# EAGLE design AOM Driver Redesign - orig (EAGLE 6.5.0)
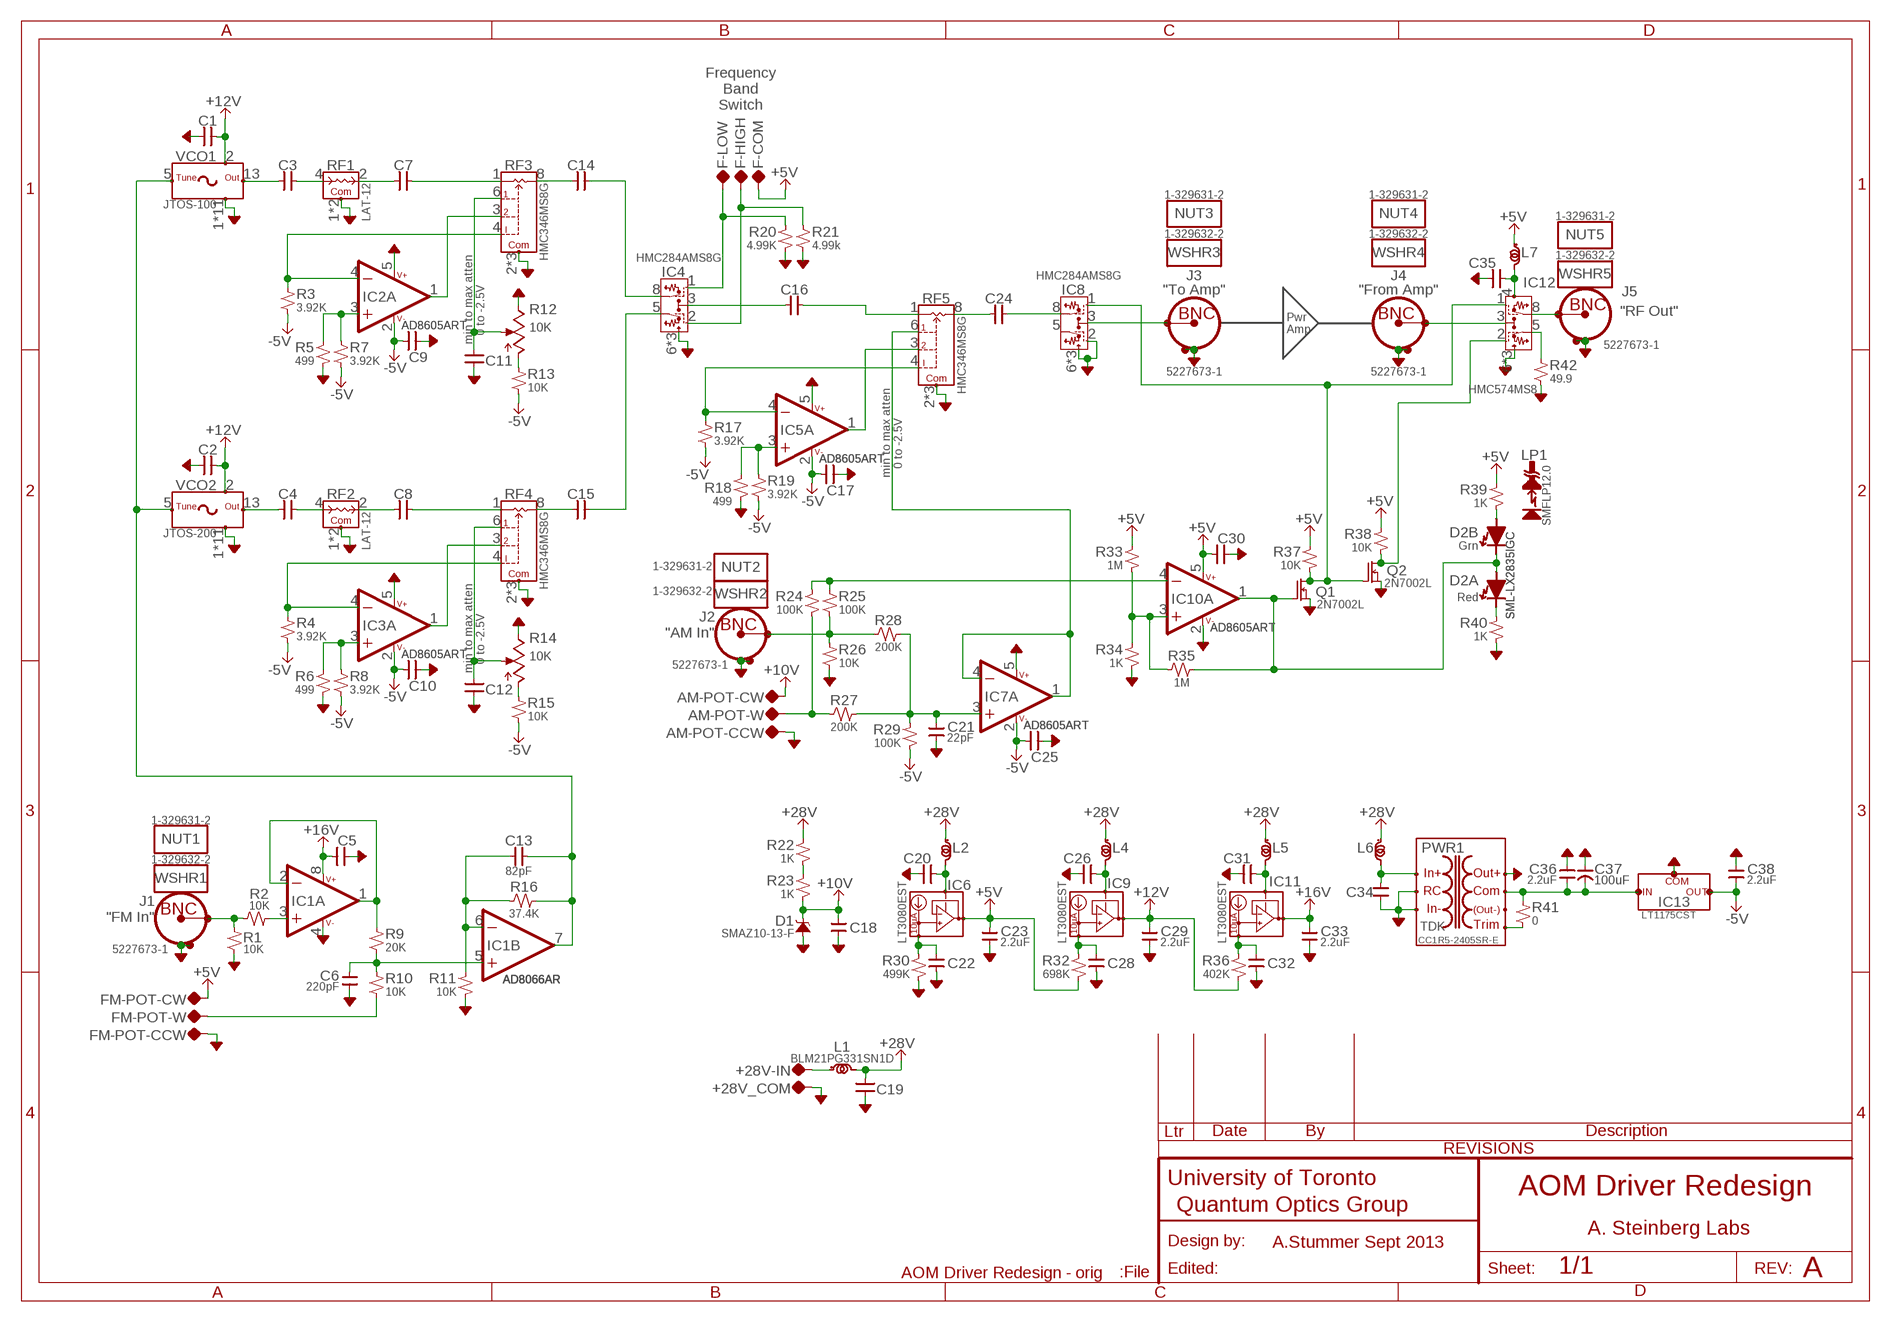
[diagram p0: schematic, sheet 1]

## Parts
+28V-IN  TP-0.042B  [TP-0.042B]
+28V_COM  TP-0.042B  [TP-0.042B]
AM-POT-CCW  TP-0.042B  [TP-0.042B]
AM-POT-CW  TP-0.042B  [TP-0.042B]
AM-POT-W  TP-0.042B  [TP-0.042B]
C1  0.1uF  CAP-H-0805  [2012(0805)]
C2  0.1uF  CAP-H-0805  [2012(0805)]
C3  0.1uF  CAP-H-0805  [2012(0805)]
C4  0.1uF  CAP-H-0805  [2012(0805)]
C5  0.1uF  CAP-H-0805  [2012(0805)]
C6  220pF  CAP-V-0805  [2012(0805)]
C7  0.1uF  CAP-H-0805  [2012(0805)]
C8  0.1uF  CAP-H-0805  [2012(0805)]
C9  0.1uF  CAP-H-0805  [2012(0805)]
C10  0.1uF  CAP-H-0805  [2012(0805)]
C11  0.1uF  CAP-H-0805  [2012(0805)]
C12  0.1uF  CAP-H-0805  [2012(0805)]
C13  82pF  CAP-H-0805  [2012(0805)]
C14  0.1uF  CAP-H-0805  [2012(0805)]
C15  0.1uF  CAP-H-0805  [2012(0805)]
C16  0.1uF  CAP-H-0805  [2012(0805)]
C17  0.1uF  CAP-H-0805  [2012(0805)]
C18  0.1uF  CAP-V-0805  [2012(0805)]
C19  0.1uF  CAP-H-0805  [2012(0805)]
C20  0.1uF  CAP-H-0805  [2012(0805)]
C21  22pF  CAP-V-0805  [2012(0805)]
C22  0.1uF  CAP-V-0805  [2012(0805)]
C23  2.2uF  CAP-V-0805  [2012(0805)]
C24  0.1uF  CAP-H-0805  [2012(0805)]
C25  0.1uF  CAP-H-0805  [2012(0805)]
C26  0.1uF  CAP-H-0805  [2012(0805)]
C28  0.1uF  CAP-V-0805  [2012(0805)]
C29  2.2uF  CAP-V-0805  [2012(0805)]
C30  0.1uF  CAP-H-0805  [2012(0805)]
C31  0.1uF  CAP-H-0805  [2012(0805)]
C32  0.1uF  CAP-V-0805  [2012(0805)]
C33  2.2uF  CAP-V-0805  [2012(0805)]
C34  0.1uF  CAP-V-0805  [2012(0805)]
C35  0.1uF  CAP-H-0805  [2012(0805)]
C36  2.2uF  CAP-V-0805  [2012(0805)]
C37  100uF  CAP-POL-EIA-7343-13  [EIA-7343]
C38  2.2uF  CAP-V-0805  [2012(0805)]
D1  SMAZ10-13-F  ZENER-EIA-A  [EIA-A(SMA)]
D2  SML-LX2835IGC  LED,DUAL_SEP-PLCC4B  [PLCC4B]
F-COM  TP-0.042"  [TP-0.042]
F-HIGH  TP-0.042"  [TP-0.042]
F-LOW  TP-0.042"  [TP-0.042]
FM-POT-CCW  TP-0.042B  [TP-0.042B]
FM-POT-CW  TP-0.042B  [TP-0.042B]
FM-POT-W  TP-0.042B  [TP-0.042B]
IC1  AD8066AR  OPAMP:AD8___(DUAL)-SOIC-8  [SOIC-8]
IC2  AD8605ART  OPAMP-SOT23-5  [SOT23-5]
IC3  AD8605ART  OPAMP-SOT23-5  [SOT23-5]
IC4  HMC284AMS8G  RF,SWITCH,SPDT#1-MSOP8GND  [MSOP8GND]
IC5  AD8605ART  OPAMP-SOT23-5  [SOT23-5]
IC6  LT3080EST  REGULATOR:LT3080(3PIN,LDO,I-SET)-SOT223  [SOT223]
IC7  AD8605ART  OPAMP-SOT23-5  [SOT23-5]
IC8  HMC284AMS8G  RF,SWITCH,SPDT#1-MSOP8GND  [MSOP8GND]
IC9  LT3080EST  REGULATOR:LT3080(3PIN,LDO,I-SET)-SOT223  [SOT223]
IC10  AD8605ART  OPAMP-SOT23-5  [SOT23-5]
IC11  LT3080EST  REGULATOR:LT3080(3PIN,LDO,I-SET)-SOT223  [SOT223]
IC12  HMC574MS8  RF,SWITCH,SPDT#2-MSOP8GND  [MSOP8GND]
IC13  LT1175CST  REGULATOR:NEG-3-TERM-SOT223  [SOT223]
J1  5227673-1  CONN:BNC-TYPE2VERT  [CONN:BNC-AMP-TYPE2VERT]
J2  5227673-1  CONN:BNC-TYPE2VERT  [CONN:BNC-AMP-TYPE2VERT]
J3  5227673-1  CONN:BNC-TYPE2VERT  [CONN:BNC-AMP-TYPE2VERT]
J4  5227673-1  CONN:BNC-TYPE2VERT  [CONN:BNC-AMP-TYPE2VERT]
J5  5227673-1  CONN:BNC-TYPE2VERT  [CONN:BNC-AMP-TYPE2VERT]
L1  BLM21PG331SN1D  INDUCTOR0805  [2012(0805)]
L2  BLM21PG331SN1D  INDUCTOR0805  [2012(0805)]
L4  BLM21PG331SN1D  INDUCTOR0805  [2012(0805)]
L5  BLM21PG331SN1D  INDUCTOR0805  [2012(0805)]
L6  BLM21PG331SN1D  INDUCTOR0805  [2012(0805)]
L7  BLM21PG331SN1D  INDUCTOR0805  [2012(0805)]
LP1  SMFLP12.0  LIGHTPIPE-BIVAR_SMFLP  [LIGHTPIPE,BIVAR_SMFLP]
NUT1  1-329631-2  MISC  [MISC]
NUT2  1-329631-2  MISC  [MISC]
NUT3  1-329631-2  MISC  [MISC]
NUT4  1-329631-2  MISC  [MISC]
NUT5  1-329631-2  MISC  [MISC]
PWR1  CC1R5-2405SR-E  DC-DC:CCP-__-E(TDK1.5-25W)-CC1R5-R-E  [DC-DC:CC1R5-XXXXX-R-E(TDK/LAMBDA)]
Q1  2N7002L  MOSFET-N-SOT23  [SOT23]
Q2  2N7002L  MOSFET-N-SOT23  [SOT23]
R1  10K  R-V-0805  [2012(0805)]
R2  10K  R-H-0805  [2012(0805)]
R3  3.92K  R-V-0805  [2012(0805)]
R4  3.92K  R-V-0805  [2012(0805)]
R5  499  R-V-0805  [2012(0805)]
R6  499  R-V-0805  [2012(0805)]
R7  3.92K  R-V-0805  [2012(0805)]
R8  3.92K  R-V-0805  [2012(0805)]
R9  20K  R-V-0805  [2012(0805)]
R10  10K  R-V-0805  [2012(0805)]
R11  10K  R-V-0805  [2012(0805)]
R12  10K  POT-BOURNS_3296Y  [BOURNS:3296Y]
R13  10K  R-V-0805  [2012(0805)]
R14  10K  POT-BOURNS_3296Y  [BOURNS:3296Y]
R15  10K  R-V-0805  [2012(0805)]
R16  37.4K  R-H-0805  [2012(0805)]
R17  3.92K  R-V-0805  [2012(0805)]
R18  499  R-V-0805  [2012(0805)]
R19  3.92K  R-V-0805  [2012(0805)]
R20  4.99K  R-V-0805  [2012(0805)]
R21  4.99k  R-V-0805  [2012(0805)]
R22  1K  R-V-0805  [2012(0805)]
R23  1K  R-V-0805  [2012(0805)]
R24  100K  R-V-0805  [2012(0805)]
R25  100K  R-V-0805  [2012(0805)]
R26  10K  R-V-0805  [2012(0805)]
R27  200K  R-H-0805  [2012(0805)]
R28  200K  R-H-0805  [2012(0805)]
R29  100K  R-V-0805  [2012(0805)]
R30  499K  R-V-0805  [2012(0805)]
R32  698K  R-V-0805  [2012(0805)]
R33  1M  R-V-0805  [2012(0805)]
R34  1K  R-V-0805  [2012(0805)]
R35  1M  R-H-0805  [2012(0805)]
R36  402K  R-V-0805  [2012(0805)]
R37  10K  R-V-0805  [2012(0805)]
R38  10K  R-V-0805  [2012(0805)]
R39  1K  R-V-0805  [2012(0805)]
R40  1K  R-V-0805  [2012(0805)]
R41  0  R-V-0805  [2012(0805)]
R42  49.9  R-V-0805  [2012(0805)]
RF1  LAT-12  RF,ATTEN#1-MINICIRCUITS_MMM168  [MINICIRCUITS_MMM168]
RF2  LAT-12  RF,ATTEN#1-MINICIRCUITS_MMM168  [MINICIRCUITS_MMM168]
RF3  HMC346MS8G  RF,ATTEN#2-MSOP8GND  [MSOP8GND]
RF4  HMC346MS8G  RF,ATTEN#2-MSOP8GND  [MSOP8GND]
RF5  HMC346MS8G  RF,ATTEN#2-MSOP8GND  [MSOP8GND]
VCO1  JTOS-100  RF,VCO#1-MINICIRCUITS_BK377  [MINICIRCUITS_BK377]
VCO2  JTOS-200  RF,VCO#1-MINICIRCUITS_BK377  [MINICIRCUITS_BK377]
WSHR1  1-329632-2  MISC  [MISC]
WSHR2  1-329632-2  MISC  [MISC]
WSHR3  1-329632-2  MISC  [MISC]
WSHR4  1-329632-2  MISC  [MISC]
WSHR5  1-329632-2  MISC  [MISC]

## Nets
+5V [Power]: C23.2 C30.2 F-COM.TP FM-POT-CW.TP IC6.2(OUT) IC6.4(OUT) IC10.5(B:V++) L7.1(A) R32.1 R33.2 R37.2 R38.2 R39.2
+10V: AM-POT-CW.TP C18.2 D1.K(C) R23.1
+12V [Power]: C1.2 C2.2 C29.2 IC9.2(OUT) IC9.4(OUT) R36.1 VCO1.2(VDD) VCO2.2(VDD)
+16V: C5.2 C33.2 IC1.8(PWR:V++) IC11.2(OUT) IC11.4(OUT)
+28V [Power]: C19.1 L1.2(B) L2.1(A) L4.1(A) L5.1(A) L6.1(A) R22.2
-5V [Power]: C9.2 C10.2 C17.2 C25.2 C38.1 IC2.2(B:V-) IC3.2(B:V-) IC5.2(B:V-) IC7.2(B:V-) IC13.1(OUT) R3.1 R4.1 R7.1 R8.1 R13.1 R15.1 R17.1 R19.1 R29.1
AGND: +28V_COM.TP AM-POT-CCW.TP C1.1 C2.1 C5.1 C6.1 C9.1 C10.1 C11.2 C12.2 C17.1 C18.1 C19.2 C20.1 C21.1 C22.1 C23.1 C25.1 C26.1 C28.1 C29.1 C30.1 C31.1 C32.1 C33.1 C34.1 C35.1 C36.2 C37.+(POS) C38.2 D1.A FM-POT-CCW.TP IC1.4(PWR:V-) IC2.5(B:V++) IC3.5(B:V++) IC4.6(COM) IC4.7(COM) IC4.PAD(COM) IC5.5(B:V++) IC7.5(B:V++) IC8.2(B) IC8.6(COM) IC8.7(COM) IC8.PAD(COM) IC10.2(B:V-) IC12.6(COM) IC12.7(COM) IC12.PAD(COM) IC13.3(COM) J1.SHIELD1 J1.SHIELD2 J2.SHIELD1 J2.SHIELD2 J3.SHIELD1 J3.SHIELD2 J4.SHIELD1 J4.SHIELD2 J5.SHIELD1 J5.SHIELD2 PWR1.+VOUT(+OUT) PWR1.-VIN(-IN) PWR1.RC Q1.2(S) Q2.2(S) R1.1 R5.1 R6.1 R11.1 R12.CW R14.CW R18.1 R20.1 R21.1 R26.1 R30.1 R34.1 R40.1 R42.1 RF1.1(COM) RF1.3(COM) RF2.1(COM) RF2.3(COM) RF3.2(COM) RF3.7(COM) RF3.PAD(COM) RF4.2(COM) RF4.7(COM) RF4.PAD(COM) RF5.2(COM) RF5.7(COM) RF5.PAD(COM) VCO1.1(COM) VCO1.3(COM) VCO1.4(COM) VCO1.6(COM) VCO1.7(COM) VCO1.8(COM) VCO1.9(COM) VCO1.10(COM) VCO1.11(COM) VCO1.12(COM) VCO1.14(COM) VCO2.1(COM) VCO2.3(COM) VCO2.4(COM) VCO2.6(COM) VCO2.7(COM) VCO2.8(COM) VCO2.9(COM) VCO2.10(COM) VCO2.11(COM) VCO2.12(COM) VCO2.14(COM)
N$1 [RF]: C3.1 VCO1.13(OUT)
N$2: +28V-IN.TP L1.1(A)
N$3 [RF]: C3.2 RF1.4(RF-IN)
N$4 [RF]: C7.1 RF1.2(RF-OUT)
N$5 [RF]: C7.2 RF3.1(RF1)
N$6: IC2.3(A:+IN) R5.2 R7.2
N$7: IC2.4(A:-IN) R3.2 RF3.4(I)
N$8: IC2.1(A:OUT) RF3.3(V2)
N$9: C11.1 R12.W RF3.6(V1)
N$10: R12.CCW R13.2
N$11: C13.2 IC1.7(B:OUT) R16.2 VCO1.5(VTUNE) VCO2.5(VTUNE)
N$12 [RF]: C4.1 VCO2.13(OUT)
N$13 [RF]: C4.2 RF2.4(RF-IN)
N$14 [RF]: C8.1 RF2.2(RF-OUT)
N$15 [RF]: C8.2 RF4.1(RF1)
N$16: IC3.3(A:+IN) R6.2 R8.2
N$17: IC3.4(A:-IN) R4.2 RF4.4(I)
N$18: IC3.1(A:OUT) RF4.3(V2)
N$19: C12.1 R14.W RF4.6(V1)
N$20: R14.CCW R15.2
N$21 [RF]: C16.2 RF5.1(RF1)
N$22 [RF]: C14.1 RF3.8(RF2)
N$23 [RF]: C15.1 RF4.8(RF2)
N$24 [RF]: C15.2 IC4.5(RF1)
N$25 [RF]: C14.2 IC4.8(RF2)
N$26 [RF]: C16.1 IC4.3(RFC)
N$27 [RF]: C24.1 RF5.8(RF2)
N$28: IC5.3(A:+IN) R18.2 R19.2
N$29: IC5.4(A:-IN) R17.2 RF5.4(I)
N$30: IC5.1(A:OUT) RF5.3(V2)
N$31: IC7.1(A:OUT) IC7.4(A:-IN) RF5.6(V1)
N$32: F-LOW.TP IC4.1(A) R20.2
N$33: F-HIGH.TP IC4.2(B) R21.2
N$34 [RF]: C24.2 IC8.8(RF2)
N$35: IC10.4(A:-IN) R24.2 R25.2
N$37: FM-POT-W.TP R10.1
N$38 [RF]: IC8.3(RFC) J3.CONDUCTOR
N$39 [RF]: IC12.8(RF2) J5.CONDUCTOR
N$40: IC12.5(RF1) R42.2
N$41: IC8.1(A) IC12.1(A) Q1.3(D) Q2.1(G) R37.1
N$42: IC12.2(B) Q2.3(D) R38.1
N$43 [RF]: IC12.3(RFC) J4.CONDUCTOR
N$44: AM-POT-W.TP R24.1 R27.1
N$45: J2.CONDUCTOR R25.1 R26.2 R28.1
N$46: C21.2 IC7.3(A:+IN) R27.2 R28.2 R29.2
N$47: D2.1(A:C) R40.2
N$48: IC10.3(A:+IN) R33.1 R34.2 R35.1
N$49: D2.4(B:A) R39.1
N$50: D2.2(A:A) D2.3(B:C) IC10.1(A:OUT) Q1.1(G) R35.2
N$51: J1.CONDUCTOR R1.2 R2.1
N$52: IC1.3(A:+IN) R2.2
N$53: IC1.1(A:OUT) IC1.2(A:-IN) R9.2
N$54: C6.2 IC1.5(B:+IN) R9.1 R10.2
N$55: C13.1 IC1.6(B:-IN) R11.2 R16.1
N$56 [Power]: C36.1 C37.-(NEG) IC13.2(VI) IC13.4(VI) PWR1.COM R41.2
N$57: C20.2 IC6.3(IN) L2.2(B)
N$58: C22.2 IC6.1(SET) R30.2
N$59: R22.1 R23.2
N$60: C31.2 IC11.3(IN) L5.2(B)
N$61: C26.2 IC9.3(IN) L4.2(B)
N$62: C28.2 IC9.1(SET) R32.2
N$63: C32.2 IC11.1(SET) R36.2
N$64: C35.2 IC12.4(VDD) L7.2(B)
N$82 [Power]: C34.2 L6.2(B) PWR1.+VIN(+IN)
N$87: PWR1.TRM(TRIM) R41.1
Unconnected: IC8.5(RF1) PWR1.-VOUT(-OUT)

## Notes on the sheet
- Frequency
  Band
  Switch
- Pwr
  Amp
- min to max atten
     0 to -2.5V
- min to max atten
     0 to -2.5V
- Grn
- Red
- min to max atten
     0 to -2.5V
- AOM Driver Redesign
- A. Steinberg Labs
- A.Stummer Sept 2013
- A

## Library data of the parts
+28V-IN +28V_COM AM-POT-CCW AM-POT-CW AM-POT-W F-COM F-HIGH F-LOW FM-POT-CCW FM-POT-CW FM-POT-W = QuantumOptics:TP: Testpoint, single pin or single socket, either SMT pad, small hole or loop style TP such as Keystone 5002K (0.042").
C1-C5 C7-C17 C19 C20 C24-C26 C30 C31 C35 = QuantumOptics:CAP-H-: Cap, SMT and Through-hole, 0402 and up.
C6 C18 C21-C23 C28 C29 C32-C34 C36 C38 = QuantumOptics:CAP-V-: Cap, SMT and Through-hole, 0402 and up.
C37 = QuantumOptics:CAP-POL-: Capacitor, Polarized, SMT 0805 and up, probably tantalum.; MFG: Panasonic; PN: EEF-UD0J101R
D1 = QuantumOptics:ZENER: Zener
D2 = QuantumOptics:LED,DUAL_SEP: Dual LED, Individual such as Lumex SML-LX2835IGC.
IC1 = QuantumOptics:OPAMP:AD8___(DUAL): AD8xxx, Analog Devices, dual opamp in SOIC-8 and MSOP-8, various versions available. AD8066, AD8656, etc. e.g. http://www.analog.com/UploadedFiles/Data_Sheets/476080131AD8655_6_a.pdf
IC2 IC3 IC5 IC7 IC10 = QuantumOptics:OPAMP: Op Amp, generic, pick the right package. e.g. AD8605: SOT-23-5, RRIO, 10MHz, Ib = 1pA, Vio < 65uV, 2.7-5.5V.
IC4 IC8 = QuantumOptics:RF,SWITCH,SPDT#1: RF Switch, non-reflective, such as Hittite HMC284
IC6 IC9 IC11 = QuantumOptics:REGULATOR:LT3080(3PIN,LDO,I-SET): LT3080, LDO, output set by single resistor, nice part, LinTech, 1A, SOT223, MSOP8, TO220. http://cds.linear.com/docs/Datasheet/3080f.pdf
IC12 = QuantumOptics:RF,SWITCH,SPDT#2: RF Switch, pseudo SPDT, such as Hittite HMC574
IC13 = QuantumOptics:REGULATOR:NEG-3-TERM: Negative 3-Pin, such as LM2990, http://www.national.com/ds/LM/LM2990.pdf
J1 = QuantumOptics:CONN:BNC: BNC PCB, horizontal or vertical, e.g. Horiz: Amp (5)227677-1, nut 1-329631-2, shoulder washer 330620, vert isolated 5227222-6, http://catalog.tycoelectronics.com/TE/bin/TE.Connect?C=1&M=BYPN&TCPN=5227222-6&RQPN=5227222-6 ...; DESC: "FM In"
J2 = QuantumOptics:CONN:BNC: BNC PCB, horizontal or vertical, e.g. Horiz: Amp (5)227677-1, nut 1-329631-2, shoulder washer 330620, vert isolated 5227222-6, http://catalog.tycoelectronics.com/TE/bin/TE.Connect?C=1&M=BYPN&TCPN=5227222-6&RQPN=5227222-6 ...; DESC: "AM In"
J3 = QuantumOptics:CONN:BNC: BNC PCB, horizontal or vertical, e.g. Horiz: Amp (5)227677-1, nut 1-329631-2, shoulder washer 330620, vert isolated 5227222-6, http://catalog.tycoelectronics.com/TE/bin/TE.Connect?C=1&M=BYPN&TCPN=5227222-6&RQPN=5227222-6 ...; DESC: "To Amp"
J4 = QuantumOptics:CONN:BNC: BNC PCB, horizontal or vertical, e.g. Horiz: Amp (5)227677-1, nut 1-329631-2, shoulder washer 330620, vert isolated 5227222-6, http://catalog.tycoelectronics.com/TE/bin/TE.Connect?C=1&M=BYPN&TCPN=5227222-6&RQPN=5227222-6 ...; DESC: "From Amp"
J5 = QuantumOptics:CONN:BNC: BNC PCB, horizontal or vertical, e.g. Horiz: Amp (5)227677-1, nut 1-329631-2, shoulder washer 330620, vert isolated 5227222-6, http://catalog.tycoelectronics.com/TE/bin/TE.Connect?C=1&M=BYPN&TCPN=5227222-6&RQPN=5227222-6 ...; DESC: "RF Out"
L1 L2 L4-L7 = QuantumOptics:INDUCTOR: Inductor, generic inductor.
LP1 = QuantumOptics:LIGHTPIPE: Lightpipe for SMT LEDs
NUT1-NUT5 WSHR1-WSHR5 = QuantumOptics:MISC: Miscellaneous Part, just a placeholder for miscellaeous parts
PWR1 = QuantumOptics:DC-DC:CCP-__-E(TDK1.5-25W): CCp-inoutsc-E, TDK DC-DC isolated, 1.5-25W, uni- or bipolar "p": 1.5, 3, 6, 10, 15, or 25W. "in": Input 05, 12, 24 or 48V. "out": Output 3.3, 5, 12, ±12 (or 24), ±15 (or30V). "s": Polarity single or dual. "c": Case horiz DIP, horiz SMD or vertical SIP. http://www.tdk.co.jp/tefe02/ea335_cc_e.pdf
Q1 Q2 = QuantumOptics:MOSFET-N: Mosfet, N-Channel, generic enhancement mode N-FET.
R1 R3-R11 R13 R15 R17-R26 R29 R30 R32-R34 R36-R42 = QuantumOptics:R-V-*: Resistor, SMT & Through-Hole, vertical symbol
R2 R16 R27 R28 R35 = QuantumOptics:R-H-*: Resistor, SMT & Through-Hole, horizontal symbol
R12 R14 = QuantumOptics:POT: Pot, regular or trimpot; PN: 3296Y-103
RF1 RF2 = QuantumOptics:RF,ATTEN#1: RF Attenuator, fixed, e.g. Minicircuits LAT-12.
RF3-RF5 = QuantumOptics:RF,ATTEN#2: Voltage Variable Attenuator with three controls, e.g. Hittite HMC346.
VCO1 VCO2 = QuantumOptics:RF,VCO#1: VCO, with tunng, such as Minicircuits JTOS-100

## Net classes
0 default: drill 0.508 mm
1 Power: width 0.4 mm, drill 0.711 mm
2 RF: width 0.4 mm, drill 0.508 mm

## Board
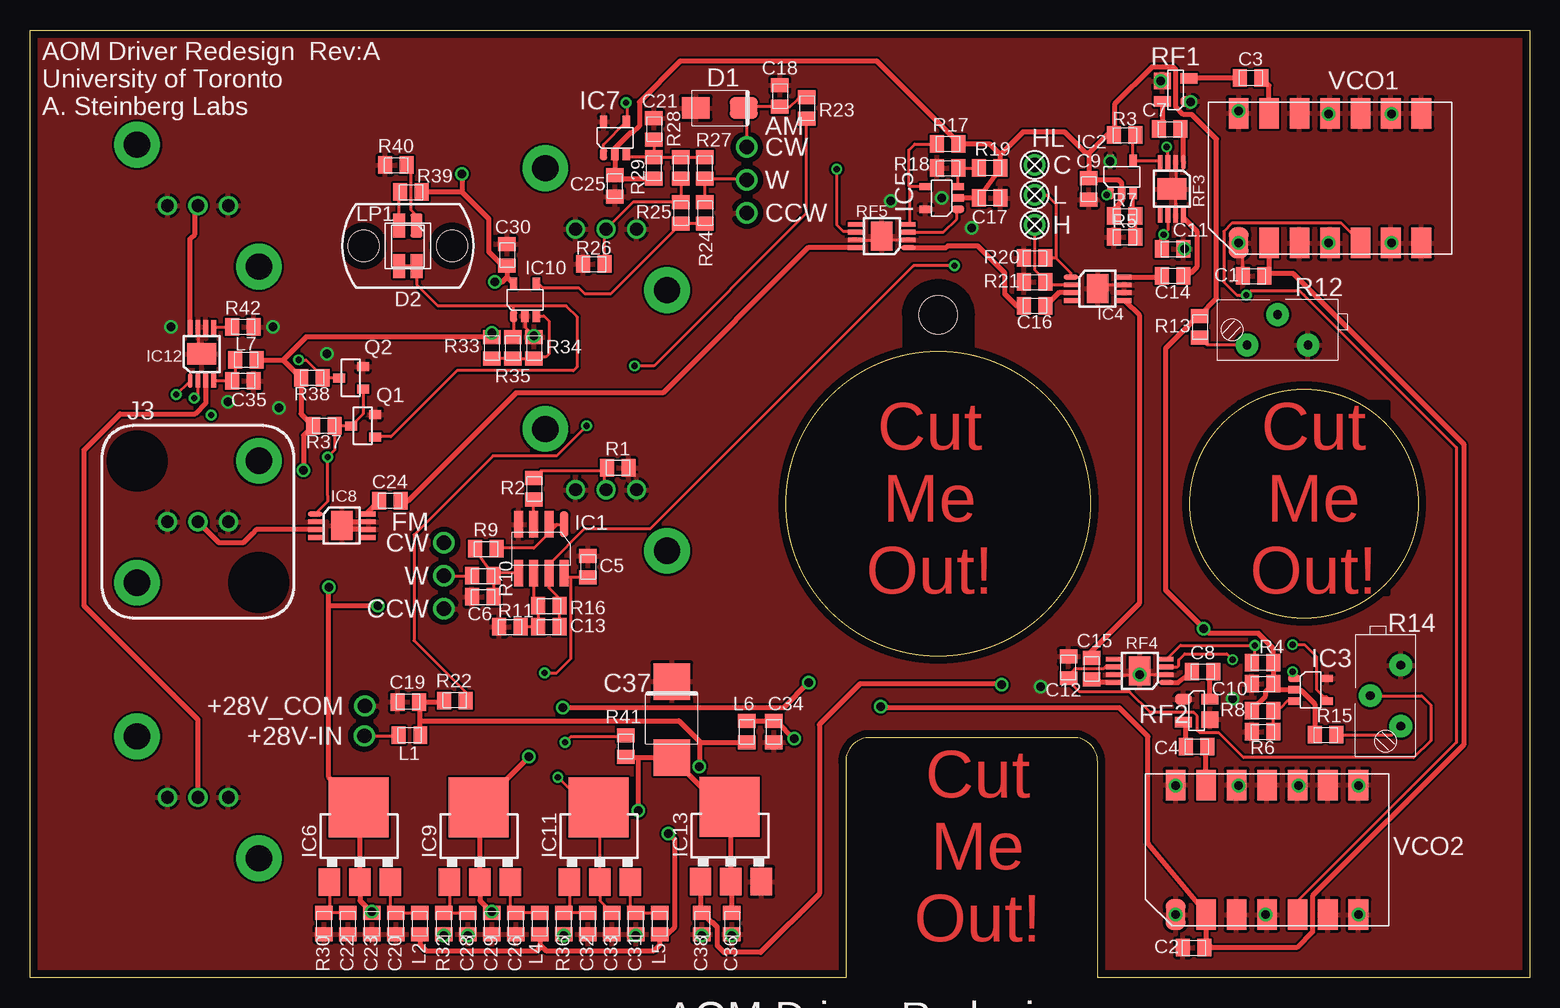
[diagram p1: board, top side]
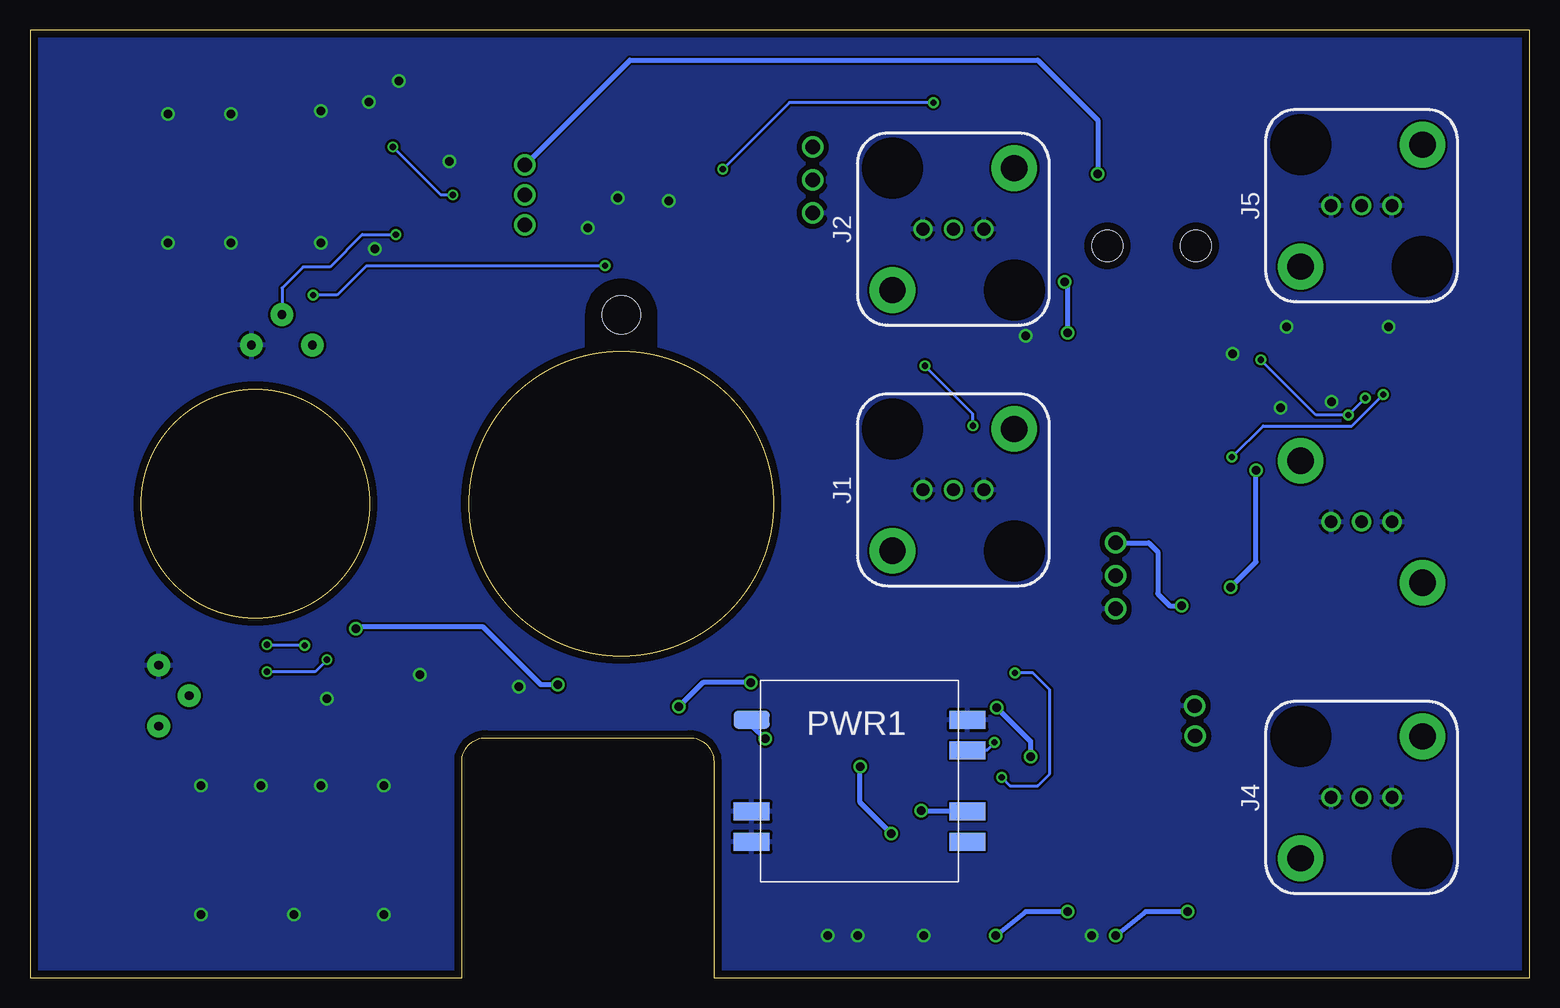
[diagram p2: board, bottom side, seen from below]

Size 125 x 79 mm. Coordinates in mm from the lower left corner, seen from the top.
Outline: 125,0 89,0 89,18 arc90 87,20 70,20 arc90 68,18 68,0 0,0 0,79 125,79 125,0
Outline: circle at 75.72,39.51 radius 12.7
Outline: circle at 106.21,39.51 radius 9.53
Copper layers (1+16): Top 0.035mm / dielectric 1.5mm / Bottom 0.035mm
Design rules "DRC standard check": minimum track width 0.18mm, minimum drill 20mil, track to track 0.18mm, track to pad 0.18mm, pad to pad 0.18mm, via to via 0.18mm, smd to smd 0mil, copper to edge 25mil, drill to drill 7mil, minimum pad ring 7mil, minimum via ring 8mil, stop-mask expansion 4mil, vias tented up to drill 0mil, thermal gap 10mil
Holes 3.17 mm at 75.72,55.25
tRestrict: area 72.7,51.8 to 78.7,55.2; 1 lines
bRestrict: area 72.7,51.8 to 78.7,55.2; 2 lines

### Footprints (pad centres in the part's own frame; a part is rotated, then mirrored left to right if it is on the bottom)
TP-0.042B = drill 1.181: TP 0,0
2012(0805) = smd 1.15 x 1.45: 1 -0.9,0; 2 0.9,0
EIA-7343 = smd 3.048 x 3.048: + 3.175,0; - -3.175,0
EIA-A(SMA) = smd 2.3 x 1.8: A -2,0; K 2,0
PLCC4B = smd 2 x 1: 1 1.7,-0.725; 2 -1.7,-0.725; 3 -1.7,0.725; 4 1.7,0.725
TP-0.042 = drill 1.181: TP 0,0
SOIC-8 = smd 0.75 x 2.2: 1 -1.27,-2.032; 2 0,-2.032; 3 1.27,-2.032; 4 2.54,-2.032; 5 2.54,2.032; 6 1.27,2.032; 7 0,2.032; 8 -1.27,2.032
SOT23-5 = smd 0.6 x 1: 1 -0.95,-1.35; 2 0,-1.35; 3 0.95,-1.35; 4 0.95,1.35; 5 -0.95,1.35
MSOP8GND = smd 0.4 x 1.2: 1 -0.65,-2.223; 2 0,-2.223; 3 0.65,-2.223; 4 1.3,-2.223; 5 1.3,2.223; 6 0.65,2.223; 7 0,2.223; 8 -0.65,2.223 | smd 2.413 x 1.778: PAD 0.325,0
SOT223 = smd 1.778 x 2.3: 1 -2.54,-2.54; 3 2.54,-2.54 | smd 1.778 x 2.286: 2 0,-2.54 | smd 5 x 5: 4 -0.1,3.7
CONN:BNC-AMP-TYPE2VERT = drill 1.067: CONDUCTOR 0,0; SHIELD1 -2.54,0; SHIELD2 2.54,0 | drill 2.184 pad 3.81: MTG1 -5.08,-5.08; MTG2 5.08,5.08
LIGHTPIPE,BIVAR_SMFLP = hole 2.578: -3.683,0; 3.683,0
DC-DC:CC1R5-XXXXX-R-E(TDK/LAMBDA) = smd 3 x 1.5: +VIN -9,5.1; +VOUT 9,5.08; -VIN -9,-5.08; -VOUT 9,-5.08; COM 9,-2.54; RC -9,-2.54; TRM 9,2.54
SOT23 = smd 0.75 x 1: 1 -0.95,-1; 2 0.95,-1; 3 0,1
BOURNS:3296Y = drill 0.711 pad 1.905: CCW 2.54,1.27; CW -2.54,1.27; W 0,-1.27
MINICIRCUITS_MMM168 = smd 0.889 x 1.397: 1 0.953,1.105; 2 0.953,-1.105; 4 -0.953,1.105 | smd 1.397 x 1.397: 3 -0.749,-1.105
MINICIRCUITS_BK377 = smd 1.651 x 2.54: 1 0,0; 2 2.54,0; 3 5.08,0; 4 7.62,0; 5 10.16,0; 6 12.7,0; 7 15.24,0; 8 15.24,10.795; 9 12.7,10.795; 10 10.16,10.795; 11 7.62,10.795; 12 5.08,10.795; 13 2.54,10.795; 14 0,10.795

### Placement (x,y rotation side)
+28V-IN  27.87,20.14 180 top
+28V_COM  27.92,22.64 180 top
AM-POT-CCW  59.75,63.75 0 top
AM-POT-CW  59.75,69.25 270 top
AM-POT-W  59.75,66.5 0 top
C1  102,58.5 0 top
C2  97,2.5 0 top
C3  101.75,75 180 top
C4  97.25,19.25 180 top
C5  46.5,34.25 270 top
C6  37.75,31.75 0 top
C7  95,70.75 0 top
C8  97.75,25.5 180 top
C9  88.25,65.75 90 top
C10  102.75,24.5 0 top
C11  95.25,60.75 0 top
C12  86.57,25.86 90 top
C13  43.25,29.25 0 top
C14  95.25,58.5 180 top
C15  88.5,25.75 90 top
C16  83.75,56 180 top
C17  80,65 180 top
C18  62.5,73.5 270 top
C19  31.54,22.96 180 top
C20  30.5,4.5 90 top
C21  52,70.75 270 top
C22  26.5,4.5 90 top
C23  28.5,4.5 90 top
C24  30,39.75 180 top
C25  48.75,66 90 top
C26  40.5,4.5 90 top
C28  36.5,4.5 90 top
C29  38.5,4.5 90 top
C30  39.75,60.25 270 top
C31  50.5,4.5 90 top
C32  46.5,4.5 90 top
C33  48.5,4.5 90 top
C34  62,20.5 90 top
C35  17.75,49.75 180 top
C36  58.5,4.5 270 top
C37  53.5,21.5 90 top
C38  56,4.5 270 top
D1  57.5,72.5 0 top
D2  31.5,61 90 top
F-COM  83.75,67.75 0 top
F-HIGH  83.75,62.75 90 top
F-LOW  83.75,65.25 180 top
FM-POT-CCW  34.5,30.75 180 top
FM-POT-CW  34.5,36.25 0 top
FM-POT-W  34.5,33.5 180 top
IC1  43.25,35.75 180 top
IC2  91,66.75 0 top
IC3  106.75,24 270 top
IC4  89,57.75 270 top
IC5  76,65 90 top
IC6  27.5,10.5 0 top
IC7  48.75,70 0 top
IC8  26,38 270 top
IC9  37.5,10.5 0 top
IC10  41.25,56.5 0 top
IC11  47.5,10.5 0 top
IC12  14,52 0 top
IC13  58.43,10.54 0 top
J1  48.03,40.66 0 bottom
J2  48.03,62.4 0 bottom
J3  14,38 0 top
J4  14,15.02 0 bottom
J5  14,64.36 0 bottom
L1  31.64,20.22 0 top
L2  32.5,4.5 90 top
L4  42.5,4.5 90 top
L5  52.5,4.5 90 top
L6  59.75,20.5 90 top
L7  18,51.5 180 top
LP1  31.5,61 0 top
NUT1  106,-2 180 top
NUT2  not placed on the board
NUT3  not placed on the board
NUT4  not placed on the board
NUT5  not placed on the board
PWR1  55.85,16.39 0 bottom
Q1  27.75,46 90 top
Q2  26.75,50 90 top
R1  49,42.5 180 top
R2  42,40.75 270 top
R3  91.25,70.25 0 top
R4  102.75,26.25 180 top
R5  91.25,61.75 0 top
R6  102.75,20.5 0 top
R7  91.25,63.5 0 top
R8  102.75,22.25 0 top
R9  38,35.75 0 top
R10  37.75,33.5 0 top
R11  40,29.25 0 top
R12  104,54 180 top
R13  97.5,54.25 270 top
R14  113,23.5 270 top
R15  108,20.25 0 top
R16  43.25,31 0 top
R17  76.5,69.5 180 top
R18  76.5,67.5 0 top
R19  80,67.5 180 top
R20  83.75,60 0 top
R21  83.75,58 0 top
R22  35.41,23.09 180 top
R23  64.75,72.5 270 top
R24  56.25,63.75 270 top
R25  54.25,63.75 270 top
R26  47,59.5 0 top
R27  56.25,67.5 90 top
R28  54.25,67.5 90 top
R29  52,67.5 90 top
R30  24.5,4.5 90 top
R32  34.5,4.5 90 top
R33  38.5,52.5 90 top
R34  42,52.5 270 top
R35  40.25,52.5 90 top
R36  44.5,4.5 90 top
R37  24.5,46 180 top
R38  23.5,50 180 top
R39  31.75,65.5 0 top
R40  30.5,67.75 0 top
R41  49.66,19.29 270 top
R42  17.75,54.25 180 top
RF1  95.5,74 270 top
RF2  97.25,22.25 90 top
RF3  95.5,65.75 180 top
RF4  92.5,25.25 90 top
RF5  71,61.5 90 top
U$47  [TITLEBLOCK_PCB]  0,-1 0 top
VCO1  100.75,61.25 0 top
VCO2  95.5,5.25 0 top
WSHR1  108,-2 0 top
WSHR2  not placed on the board
WSHR3  not placed on the board
WSHR4  not placed on the board
WSHR5  not placed on the board

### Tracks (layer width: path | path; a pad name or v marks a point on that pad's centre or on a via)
+5V  (via drill 0.71)
  Top 0.4: 39.75,58.4 C30.2 39.4,59.35 38.25,60.5 38.25,63.25 36,65.5 | 39.75,58.4 IC10.5 | 36,65.5 R39.2 | L7.1 21.1,51.5 | 21.1,51.5 R38.2 22.6,47 R37.2 22.8,45.2 v22.8,42.3 | 21.1,51.5 23,53.4 R33.2 v38.5,53.75 | 24.9,31 24.9,16.7 IC6.4 27.5,14.1 IC6.2 27.5,6.4 C23.2 v28.5,5.5 28.5,5.75 | v34.5,3.5 R32.1 | v38.75,58 39.35,58 39.75,58.4 | v36,67 36,65.5 | v29,31 24.9,31 | 24.9,31 v24.9,32.55
  Bottom 0.4: FM-POT-CW.TP 31.75,36.25 31,35.5 31,32 30,31 v29,31 | v28.5,5.5 32,5.5 v34.5,3.5 | v38.5,53.75 38.5,57.75 v38.75,58 | F-COM.TP 75,76.5 41,76.5 36,71.5 v36,67 | v22.8,42.3 22.8,34.65 v24.9,32.55
+10V
  Top 0.254: R23.1 64.6,73.25 64,73.25 63.35,72.6 C18.2 59.6,72.6 D1.K 59.75,72.25 AM-POT-CW.TP
+12V  (via drill 0.71)
  Top 0.4: VCO1.2 103.29,58.89 C1.2 103.1,58.7 105.3,58.7 119.5,44.5 119.5,19.4 106.9,6.8 106.9,3.8 105.6,2.5 98.54,2.5 98.04,3 | 98.04,3 VCO2.2 98,5.4 93.2,11.2 93.2,20.1 90.8,22.5 71,22.5 v70.9,22.6 | 98.04,3 98.04,2.64 C2.2 | v44.4,22.5 62.8,22.5 v64.9,24.6 | v44.5,3.5 R36.1 | v38.5,5.5 C29.2 37.5,6.4 IC9.2 37.5,14.1 IC9.4 v41.6,18.4
  Bottom 0.4: v38.5,5.5 42,5.5 v44.5,3.5 | v44.4,22.5 41.6,19.7 v41.6,18.4 | v64.9,24.6 68.9,24.6 v70.9,22.6
+16V  (via drill 0.51)
  Top 0.254: C33.2 47.5,6.4 IC11.2 47.5,14.1 IC11.4 47.4,14.3 46.4,14.3 v44,16.7 | C5.2 45.1,33.35 | 45.1,33.35 44.89,33.35 IC1.8 | 45.1,33.35 45.1,26.6 43.9,25.4 v42.9,25.4
  Bottom 0.254: v44,16.7 43.3,16 41,16 40,17 40,24 41.4,25.4 v42.9,25.4
+28V  (via drill 0.71)
  Top 0.4: L2.1 32.5,2.75 33,2.25 42.25,2.25 42.5,2.5 42.5,2.75 | L4.1 42.5,2.75 | 42.5,2.75 43,2.25 52,2.25 52.5,2.75 L5.1 53.1,3.6 53.75,4.25 53.75,11.55 53.65,11.55 v53.2,12 | L1.2 32.54,21.4 | 32.54,21.4 32.54,22.86 C19.1 34.38,22.96 R22.2 | 55.9,19.6 L6.1 | 55.9,19.6 54.1,21.4 32.54,21.4 | v55.8,17.6 55.8,19.5 55.9,19.6
  Bottom 0.4: v53.2,12 55.8,14.6 v55.8,17.6
-5V  (via drill 0.71)
  Top 0.4: R8.1 101.85,22.35 103,23.5 103,23.85 C10.2 | C10.2 R4.1 103.6,26.4 103.6,27.5 102.4,28.7 98.3,28.7 97.9,29.1 v97.85,29.1 94.65,32.3 94.65,52.45 97.4,55.2 R13.1 97.5,55.2 98.9,56.6 98.9,69.9 96.85,71.95 96.15,71.95 95.5,72.6 95.5,75.7 95.3,75.9 93.5,75.9 90.4,72.8 90.4,70.4 R3.1 89.75,70.25 88.25,68.75 | C10.2 104.15,24 IC3.2 105.5,23.9 106,23.9 107.1,22.8 R15.1 | IC13.1 55.89,5.51 C38.1 56.8,4.6 56.9,4.6 57.3,4.2 57.3,2.65 57.85,2.1 60.9,2.1 65.8,7 65.8,21.1 69.2,24.5 80.9,24.5 v81,24.4 | R7.1 90.5,63.65 90.5,64.25 91,64.75 IC2.2 91,66.25 90.75,66.5 88.65,66.5 C9.2 88.25,68.75 | 80.88,68.62 80.9,68.6 R19.1 C17.2 IC5.2 | 80.88,68.62 80,69.5 R17.1 77.4,69.6 70.6,76.4 54.2,76.4 50.8,73 50.8,71 50.2,70.4 50,70.4 48.8,69.2 48.8,68.8 IC7.2 48.8,68.6 48.8,66.9 C25.2 48.9,66.8 49.1,66.6 R29.1 | 88.25,68.75 88,68.75 86.25,70.5 82.75,70.5 80.88,68.62
  Bottom 0.4: v81,24.4 82.4,24.4 87.25,29.25 97.7,29.25 v97.85,29.1
AGND  (via drill 0.71)
  Top 0.18: 26.32,37.35 IC8.PAD | IC8.7 28,38
  Top 0.254: IC12.7 14,52.33 IC12.PAD | IC4.7 89.33,57.75 IC4.PAD | RF4.2 92.83,25.25 RF4.PAD 92.17,25.25 RF4.7 | RF3.7 95.5,65.42 RF3.PAD 95.5,66.08 RF3.2 | 46.6,3.6 C32.1 | RF5.7 70.67,61.5 RF5.PAD 71.33,61.5 RF5.2 | IC10.2 41.25,54.25 v42,53.5 | C1.1 101.1,60.9 VCO1.1
  Top 0.4: IC8.6 26.32,37.35 | 28,38 26.25,38
  other vias: 71.75,64.75 76,65 78.5,62.5 20.25,54.25 11.75,54.25 16.5,48 20.75,47.5 24.75,52 36.5,3.5 50.5,3.5 58.5,3.5 56,3.5 94.25,74.75 96.75,73 84.25,24.25 92.5,25.25 100.25,23.25 95.5,16 96.25,60.75 100.75,61.25 113.5,61.25 108.25,61.25 108.25,72 113.5,72 100.75,72.25 100.75,16 105.75,16 110.75,16 110.75,5.25 103,5.25 95.5,5.25 90.05,68.05
  pour Bottom: 0,0 0,79 125,79 125,0
  pour Top: 0,0 0,79 125,79 125,0
N$1
  Top 0.4: VCO1.13 103.29,74.36 C3.1
N$2
  Top 0.254: +28V-IN.TP 30.66,20.14 L1.1
N$3
  Top 0.4: C3.2 96.65,75 RF1.4
N$4
  Top 0.4: RF1.2 94.39,70.8 C7.1
N$5
  Top 0.4: RF3.1 96.15,70.25 C7.2
N$6
  Top 0.254: IC2.3 91.95,63.7 R7.2 R5.2
N$7
  Top 0.254: R3.2 91.95,70.05 IC2.4 94.07,68.1 RF3.4
N$8  (via drill 0.51)
  Top 0.254: RF3.3 94.85,68.9 v94.75,69.25 | v89.75,65.25 89.75,65.1 IC2.1
  Bottom 0.254: v89.75,65.25 90.75,65.25 v94.75,69.25
N$9  (via drill 0.51)
  Top 0.254: C11.1 94.25,60.85 94.25,61.7 v94.5,61.95 94.85,62.3 RF3.6
  Bottom 0.254: v94.5,61.95 97.3,61.95 100,59.25 102.25,59.25 104,57.5 R12.W 104,55.3
N$10
  Top 0.254: R12.CCW 98.12,52.73 R13.2
N$11  (via drill 0.51)
  Top 0.254: C13.2 R16.2 44.25,31.1 44.25,31.5 43.25,32.5 IC1.7 43.3,33.8 43.3,34.5 46.2,37.4 51.7,37.4 73.65,59.35 v77.05,59.35 | VCO2.5 105.7,5.3 105.7,6.4 118.9,19.6 118.9,44.2 106.2,56.9 105.85,57.25 101.75,57.25 v101.4,56.9 100.6,56.9 99.5,58 99.5,62.2 100.2,62.9 109.3,62.9 110.9,61.3 VCO1.5
  Bottom 0.254: v77.05,59.35 96.95,59.35 99.4,56.9 v101.4,56.9
N$12
  Top 0.4: VCO2.13 98.04,19.14 C4.1
N$13
  Top 0.4: C4.2 96.35,21.09 RF2.4
N$14
  Top 0.4: RF2.2 98.36,25.45 C8.1
N$15
  Top 0.4: RF4.1 95.7,24.6 C8.2
N$16
  Top 0.254: R6.2 R8.2 103.9,22.5 104.25,22.5 104.8,23.05 IC3.3
N$17  (via drill 0.51)
  Top 0.254: IC3.4 108.1,23.4 107.85,23.4 107.25,24 107.25,26.75 106.25,27.75 v105.25,27.75 | RF4.4 94.8,26.6 95.9,27.7 v102.1,27.7 102.1,26.5 R4.2 102,26.6
  Bottom 0.254: v105.25,27.75 102.15,27.75 v102.1,27.7
N$18  (via drill 0.51)
  Top 0.254: RF4.3 95.65,25.9 95.75,26 95.75,26.5 96.25,27 99.75,27 v100.25,26.5 | v105.25,25.5 105.4,25.35 IC3.1
  Bottom 0.254: v100.25,26.5 101.25,25.5 v105.25,25.5
N$19
  Top 0.254: RF4.6 89.65,25.9 89.5,25.75 87.1,25.75 86.57,25.22 C12.1 86.57,24.73 87.47,23.83 91.66,23.83 93.39,22.1 97,22.1 97.3,21.8 97.3,20.6 97.5,20.4 99.1,20.4 101.15,18.35 115.35,18.35 116.75,19.75 116.75,22.75 116,23.5 R14.W
N$20
  Top 0.254: R15.2 113.56,20.25 R14.CCW
N$21
  Top 0.4: C16.2 82.25,56 81.25,57 81.25,58.75 79,61 76.5,61 76.35,60.85 RF5.1
N$22
  Top 0.4: RF3.8 96.15,63.35 97.25,62.25 97.25,59.25 96.75,58.75 96.4,58.75 C14.1
N$23
  Top 0.4: RF4.8 88.5,24.6 C15.1
N$24
  Top 0.4: C15.2 88.25,27 92.5,31.25 92.5,55.17 IC4.5
N$25
  Top 0.4: IC4.8 94.25,58.4 C14.2
N$26
  Top 0.4: IC4.3 85.75,57.1 C16.1
N$27
  Top 0.4: RF5.8 64.85,60.85 52.75,48.75 40.5,48.75 31.5,39.75 C24.1
N$28
  Top 0.254: IC5.3 77.35,67.45 R18.2 R19.2
N$29
  Top 0.254: IC5.4 73.3,65.95 | 73.3,65.95 73.25,66 73.25,69 73.75,69.5 R17.2 | 73.3,65.95 73.3,62.88 RF5.4
N$30
  Top 0.254: RF5.3 76.15,62.15 77.25,63.25 77.25,63.95 IC5.1
N$31  (via drill 0.51)
  Top 0.254: IC7.1 47.8,69.45 IC7.4 49.8,71.4 49.8,72.85 v49.7,72.95 | RF5.6 68.7,62.2 67.8,62.2 67.25,62.75 v67.25,67.4
  Bottom 0.254: v49.7,72.95 61.7,72.95 v67.25,67.4
N$32
  Top 0.254: IC4.1 86.78,58.72 85.5,60 | 85.5,60 R20.2 | F-LOW.TP 84.75,65.25 85.5,64.5 85.5,60
N$33
  Top 0.254: IC4.2 85.15,57.75 R21.2 84.65,58.1 83.75,59 F-HIGH.TP
N$34
  Top 0.4: IC8.8 28.22,38.87 C24.2
N$35
  Top 0.254: 42.2,57.9 IC10.4 42.4,57.85 42.75,57.5 45.75,57.5 46.25,57 48.4,57 R25.2 54.3,62.9 56.2,62.9 R24.2
N$37
  Top 0.254: FM-POT-W.TP R10.1
N$38
  Top 0.4: J3.CONDUCTOR 15.75,36.25 17.75,36.25 18.5,37 18.85,37.35 IC8.3
N$39
  Top 0.4: IC12.8 13.35,61.6 13.75,62 13.75,64.11 J5.CONDUCTOR
N$40
  Top 0.254: IC12.5 16.82,54.22 R42.2
N$41  (via drill 0.51)
  Top 0.254: Q2.1 27.75,47 Q1.3 R37.1 25.4,44 v24.8,43.4 24.8,40.2 24.8,39.67 IC8.1 | v12.2,48.6 13.3,49.7 IC12.1
  Bottom 0.254: v12.2,48.6 14.8,46 22.2,46 v24.8,43.4
N$42  (via drill 0.51)
  Top 0.254: Q2.3 R38.1 24.4,50.1 23,51.5 v22.4,51.5 | IC12.2 14,48.6 v13.7,48.3
  Bottom 0.254: v13.7,48.3 v15.1,46.9 17.8,46.9 v22.4,51.5
N$43
  Top 0.4: J4.CONDUCTOR 14,21.5 4.5,31 4.5,44 7.5,47 13.75,47 14.65,47.9 IC12.3
N$44
  Top 0.254: R24.1 R27.1 59.65,66.6 AM-POT-W.TP
N$45
  Top 0.254: R28.1 R25.1 50.28,64.65 J2.CONDUCTOR 47.9,62.27 R26.2
N$46
  Top 0.254: C21.2 R29.2 | R29.2 49.95,68.4 IC7.3 | R29.2 R28.2 R27.2
N$47
  Top 0.254: D2.1 32.23,63.52 31.75,64 31.75,67.4 R40.2
N$48
  Top 0.254: R33.1 R35.1 R34.2 42.15,51.75 43,51.75 43.25,52 43.25,54.75 42.85,55.15 IC10.3
N$49
  Top 0.254: D2.4 30.77,65.42 R39.1
N$50
  Top 0.254: R35.2 40.3,53.45 IC10.1 40.3,55.95 40.25,56 | D2.3 D2.2 32.25,59.27 32.25,57.75 34,56 40.25,56 | Q1.1 28.8,45.1 30.1,45.1 35.6,50.6 45.3,50.6 45.6,50.9 45.6,55.1 44.7,56 40.25,56
N$51
  Top 0.254: 47.85,42.25 42.6,42.25 R2.1 | 47.85,42.25 R1.2 | 47.85,42.25 47.85,40.84 J1.CONDUCTOR
N$52
  Top 0.254: IC1.3 41.98,39.83 R2.2
N$53
  Top 0.254: IC1.2 43.9,37.78 | 43.9,37.78 IC1.1 | R9.2 38.9,35.8 42,35.8 43.9,37.7 43.9,37.78
N$54
  Top 0.254: IC1.5 38.87,33.72 R10.2 | R10.2 C6.2 | R9.1 R10.2
N$55
  Top 0.254: IC1.6 41.98,31.77 42.25,31.5 42.25,31.1 R16.1 C13.1 R11.2
N$56  (via drill 0.71)
  Top 0.4: 50.7,18.32 C37.- 57.59,14.24 IC13.4 58.43,14.14 IC13.2 58.5,7.93 C36.1 | 50.7,18.32 49.73,18.32 R41.2 | 50.7,18.32 v50.7,13.9
  Bottom 0.4: v50.7,13.9 46.9,13.9 PWR1.COM
N$57
  Top 0.254: IC6.3 30.04,5.86 C20.2 L2.2
N$58
  Top 0.254: C22.2 25,5.4 | 25,5.4 R30.2 | IC6.1 24.96,5.44 25,5.4
N$59  (via drill 0.51)
  Top 0.254: v46.4,46 43.9,43.5 38.6,43.5 32,36.9 32,28.1 36.3,23.8 R22.1 | R23.2 64.7,71.6 64.7,63.7 52,51 v50.4,51
  Bottom 0.254: v46.4,46 46.4,47 v50.4,51
N$60
  Top 0.254: IC11.3 50.04,5.86 C31.2 L5.2
N$61
  Top 0.254: IC9.3 40.04,5.86 C26.2 L4.2
N$62
  Top 0.254: R32.2 35,5.4 | 35,5.4 C28.2 | IC9.1 34.96,5.44 35,5.4
N$63
  Top 0.254: C32.2 45,5.4 | 45,5.4 R36.2 | IC11.1 44.96,5.44 45,5.4
N$64
  Top 0.254: L7.2 17.1,50 C35.2 16.82,49.78 IC12.4
N$82  (via drill 0.71)
  Top 0.4: L6.2 C34.2 62.1,21.3 62.3,21.3 v63.7,19.9
  Bottom 0.4: v63.7,19.9 64.8,21 64.8,21.4 PWR1.+VIN
N$87  (via drill 0.51)
  Top 0.254: v44.6,19.6 45.1,20.1 49.6,20.1 R41.1
  Bottom 0.254: v44.6,19.6 45.2,19 46.8,19 PWR1.TRM

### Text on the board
Top: Cut / Me / Out! | Cut / Me / Out! | Cut / Me / Out!
tNames: AOM Driver Redesign Rev:A / University of Toronto / A. Steinberg Labs | AM | HL | CW | C | W | L | CCW | H | FM | CW | W | CCW | AOM Driver Redesign / A. Steinberg Labs | A | 0.18mm (7m") | 0.4mm | 0.18mm(7m") | 0.1mm | 0.25mm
